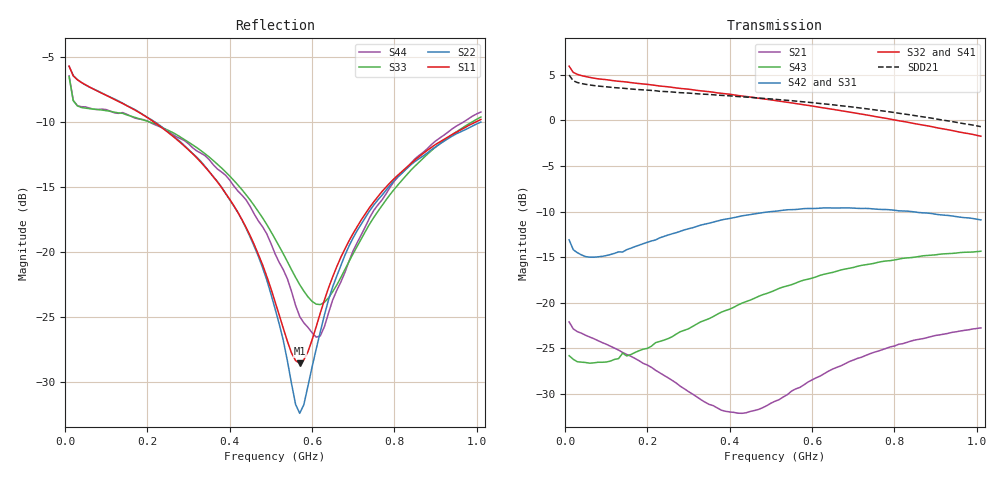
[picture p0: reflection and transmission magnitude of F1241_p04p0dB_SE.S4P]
! Integrated Device Technology
! Corporate Headquarters
! 6024 Silver Creek Valley Road
! San Jose, CA 95138  USA
! Phone:  1-408-284-8200
! Toll Free:  1-800-223-1366
! Webpage:  http://www.idt.com/
! Timing and RF Division
! 515 Groton Road, Suite 102
! Westford, MA 01886-6024
! Device:  F1241
! Description: Dual Intermediate Frequency Digital Variable Gain Amplifier
! Frequency:  10.0 -  500.00 MHz
! Package:  5x5 mm QFN Plastic Package: 32 pin
! Ports:  8 RF, 20 DC
!  Pin  1  = GA3  Pin 17  = RF OUT_B+
!  Pin  2  = GA4  Pin 18  = RF OUT_B-
!  Pin  3  = GA5  Pin 19  = STBY_B
!  Pin  4  = ISET_A  Pin 20  = Ground
!  Pin  5  = ISET_B  Pin 21  = Ground
!  Pin  6  = GB5  Pin 22  = STB_A
!  Pin  7  = GB4  Pin 23  = RF OUT_A-  = Port 4
!  Pin  8  = GB3  Pin 24  = RF OUT_A+  = Port 3
!  Pin  9  = GB2  Pin 25  = NO CONNECT
!  Pin 10  = GB1  Pin 26  = NO CONNECT
!  Pin 11  = RF IN_B+  Pin 27  = VCC
!  Pin 12  = RF IN_B-  Pin 28  = Ground
!  Pin 13  = Ground  Pin 29  = RF IN_A-  = Port 2
!  Pin 14  = VCC  Pin 30  = RF IN_A+  = Port 1
!  Pin 15  = NO CONNECT  Pin 31  = GA1
!  Pin 16  = NO CONNECT  Pin 32  = GA2
! State:  16
! Gain State:  4.0 dB
! Voltages:  Vcc = +5.00 Volts  Icc approximately 160.0 mA or 80 mA per channel.
! Data:  The device was measured on a custom evaluation board which has
!  individual transmission lines to the RF pins.  Data was collected
!  using a calibrated network analyzer.  The evaluation board was
!  de-embedded using a port reference technique.
!  The reference plane is the edge of the package pin.
!  Only Channel A was measured.
!  This data is in single-ended operation.  If your needs are balanced
!  or differential S-parameters then this file needs to be used a
!  linear simulator.
! Misc:  Lot Code  160028MY
!  Action Tracker AT004
! Date Measured:  2014-08-14
! Date:  2014-08-28  MJV
! Note:
!  Integrated Device Technology supplies this data as a sample of measured
!  data at the package pin for this product.  Your particular data for this
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# Hz S dB R 50
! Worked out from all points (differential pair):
!   101 points, 10 MHz to 1.01 GHz, reference 50 ohm
!   strongest paths, dB at 10 MHz, 260 MHz, 510 MHz, 760 MHz, 1.01 GHz:
!     S32: 6.0, 3.6, 2.2, 0.4, -1.7
!     S41: 6.0, 3.6, 2.1, 0.2, -1.9
!     S42: -13.1, -12.4, -10.0, -9.8, -10.9
!     S31: -13.1, -12.4, -10.0, -9.8, -11.0
!     S43: -25.8, -23.8, -18.6, -15.6, -14.4
!     S21: -22.1, -28.5, -30.8, -25.3, -22.8
!   taken as a pair (ports 2,1 in; 3,4 out), SDD21 dB: 5.0, 3.1, 2.3, 1.1, -0.7
!   lowest |S11| = -28.6 dB at 570 MHz (marker M1), VSWR 1.08, Z = 47.1 - j2.14 ohm
!   |S11| at or under -10 dB: 214.6 MHz to 999.2 MHz (784.6 MHz wide, 129 % of centre)
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1e7  -5.73 -16.1  -22.09 -19.3  -41.12 3.8  -18.86 12.9
     -22.12 -19.3  -5.73 -15.9  -18.88 12.6  -41.14 3.5
     -13.09 160.6  5.96 173.4  -6.55 -29.3  -25.92 -174.4
     5.99 173.4  -13.11 160.7  -25.83 -174.6  -6.48 -29.3
2.2e8  -10.12 -32.2  -27.45 -24.8  -36.18 36.9  -19.35 -14.4
       -27.43 -25.8  -10.06 -30.1  -19.35 -14.3  -36.24 35.7
       -13.10 83.4  3.85 143.1  -10.18 -22.6  -24.54 139.2
       3.84 142.5  -13.12 83.6  -24.40 139.3  -10.26 -21.3
3.8e8  -15.06 -50.6  -31.50 -5.6  -32.71 31.9  -19.25 -24.1
       -31.82 -7.3  -15.03 -46.2  -19.18 -23.7  -32.72 30.4
       -10.97 43.4  2.98 121.3  -13.56 -40.1  -21.40 114.5
       2.94 120.4  -10.92 43.0  -21.04 114.0  -13.87 -37.6
5.7e8  -28.60 -142.3  -28.81 30.2  -30.10 21.3  -19.20 -37.9
       -29.32 31.5  -32.45 -136.2  -18.98 -37.5  -30.07 18.7
       -9.78 5.8  1.79 96.9  -22.54 -93.1  -18.04 87.3
       1.70 95.8  -9.73 4.9  -17.68 86.9  -25.00 -91.5
6.2e8  -24.73 165.0  -27.66 32.1  -29.56 18.0  -19.25 -41.9
       -28.06 34.1  -26.18 157.0  -18.99 -41.5  -29.53 15.4
       -9.70 -3.0  1.43 90.8  -24.08 -132.6  -17.36 80.4
       1.34 89.7  -9.63 -4.1  -17.00 80.0  -26.50 -148.0
7.1e8  -18.06 138.3  -25.97 31.7  -28.71 11.9  -19.41 -49.0
       -26.13 34.0  -18.36 134.2  -19.08 -48.6  -28.70 8.8
       -9.73 -17.5  0.77 80.2  -19.57 172.1  -16.35 68.3
       0.65 79.0  -9.65 -19.1  -16.02 67.9  -19.29 159.6
1.01e9  -9.83 116.1  -22.89 19.7  -26.79 -10.4  -20.63 -70.8
        -22.77 21.2  -10.03 115.5  -20.04 -70.9  -26.78 -14.2
        -11.05 -55.7  -1.73 48.4  -9.64 132.3  -14.69 33.4
        -1.93 47.5  -10.92 -58.6  -14.36 32.9  -9.26 128.2
